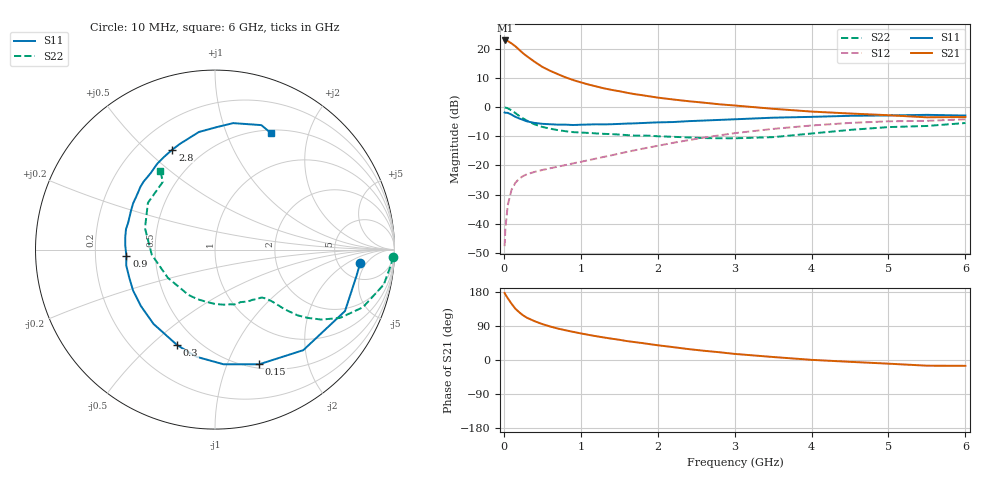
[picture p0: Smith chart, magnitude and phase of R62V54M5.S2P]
! SIEMENS Small Signal Semiconductors
! BFR193
! Si NPN RF Bipolar Junction Transistor in SOT23
! VCE = 2.5 V  IC = 4.5 mA
! Common Emitter S-Parameters:  May  1996
# GHz  S  MA  R  50
!  f  S11  S21  S12  S22
! GHz  MAG  ANG  MAG  ANG  MAG  ANG  MAG  ANG
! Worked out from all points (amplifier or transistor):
!   36 points, 10 MHz to 6 GHz, reference 50 ohm
!   highest |S21| = 22.9 dB at 20 MHz (marker M1)
!   |S21| within 3 dB of that: start of sweep to 191.4 MHz
!   unconditionally stable (mu >= 1): 899.6 MHz to 2.021 GHz
!   at 250 MHz: K = 0.40, MSG = 21.1 dB, |S12| = -23.6 dB
!   at 1.4 GHz: K = 1.07, MAG = 9.6 dB, |S12| = -16.5 dB
!   at 6 GHz: K = 0.97, MSG = 0.4 dB, |S12| = -4.1 dB
!   S11 on the Smith chart (normalised r, x): 10 MHz: 8.12, -3.52; 150 MHz: 0.54, -1.31; 300 MHz: 0.38, -0.61; 900 MHz: 0.34, -0.03; 2.8 GHz: 0.34, +0.60; 6 GHz: 0.54, +1.46
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0.01  0.8125 -5.2  13.91 176.9  0.0041 88.0  0.9923 -2.3
0.02  0.8017 -10.6  14.04 173.0  0.0082 83.9  0.9855 -4.7
0.05  0.8012 -25.3  13.74 163.3  0.0205 77.6  0.9603 -11.7
0.1  0.7456 -48.7  12.49 148.5  0.0383 66.7  0.8848 -21.3
0.15  0.6849 -68.9  11.13 135.3  0.0503 58.5  0.7933 -28.7
0.2  0.6408 -85.7  9.706 125.9  0.0593 53.3  0.7099 -33.3
0.25  0.606 -99.8  8.453 117.9  0.0657 49.2  0.6432 -36.3
0.3  0.5724 -111.6  7.516 111.5  0.0706 47.2  0.5888 -38.5
0.4  0.5374 -129.6  6.034 102.4  0.0774 45.3  0.5079 -40.7
0.5  0.5189 -142.8  4.937 94.8  0.0835 45.2  0.4595 -41.5
0.6  0.5102 -153.5  4.237 88.5  0.0893 46.1  0.4286 -42.3
0.7  0.5025 -162.3  3.711 83.1  0.0952 47.8  0.4049 -43.3
0.9  0.4948 -176.1  2.934 74.3  0.1084 51.2  0.3736 -45.6
1.1  0.5047 172.3  2.456 66.4  0.123 54.0  0.362 -49.2
1.3  0.5066 162.8  2.113 59.5  0.1403 56.2  0.3488 -53.4
1.6  0.524 150.5  1.774 49.9  0.1707 58.2  0.3318 -61.3
2.2  0.5565 130.2  1.359 34.0  0.2446 57.2  0.3103 -81.4
2.8  0.6057 113.1  1.124 20.5  0.3287 51.2  0.293 -109.4
3.5  0.6613 97.8  0.94 7.9  0.4246 40.1  0.3062 -149.2
4.5  0.7119 81.8  0.78 -4.8  0.5376 23.1  0.4079 163.0
5.5  0.74 69.6  0.671 -15.0  0.5836 5.7  0.4765 127.6
6  0.7194 64.1  0.679 -15.4  0.6204 0.7  0.5356 124.7
